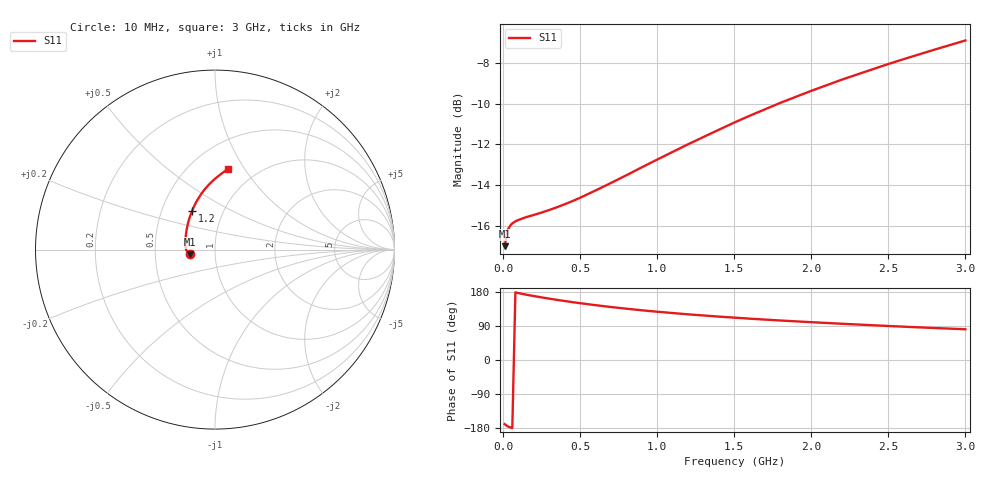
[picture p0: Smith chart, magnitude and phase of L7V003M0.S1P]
! SIEMENS Small Signal Semiconductors
! BAR14-1
! Si PIN Diode in SOT23
! IF = 3 mA
! S-Parameters:  July  1992
# GHz  S  MA  R  50
!  f  S11
! GHz  MAG  ANG
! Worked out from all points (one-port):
!   31 points, 10 MHz to 3 GHz, reference 50 ohm
!   lowest |S11| = -17.0 dB at 10 MHz (marker M1), VSWR 1.33, Z = 37.8 - j2.06 ohm
!   |S11| at or under -10 dB: start of sweep to 1.787 GHz
!   S11 on the Smith chart (normalised r, x): 10 MHz: 0.76, -0.04; 1.2 GHz: 0.71, +0.33; 3 GHz: 0.75, +0.84
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0.01  0.141 -169.1
0.03  0.1548 -175.3
0.05  0.159 -178.3
0.06  0.1604 -179.5
0.08  0.1623 178.4
0.1  0.1636 176.6
0.15  0.1662 172.4
0.2  0.1683 168.7
0.3  0.1731 161.9
0.35  0.1758 158.7
0.4  0.1788 155.7
0.5  0.1855 149.9
0.6  0.1933 144.7
0.7  0.2017 139.8
0.8  0.2107 135.4
0.9  0.2204 131.2
1  0.2303 127.4
1.2  0.2511 120.5
1.5  0.284 111.8
1.6  0.2952 109.1
1.8  0.3177 104.2
2  0.34 99.8
2.2  0.3624 95.6
2.4  0.3844 91.7
2.5  0.3958 89.8
2.6  0.4069 87.9
2.8  0.4294 84.4
3  0.4523 81.1
